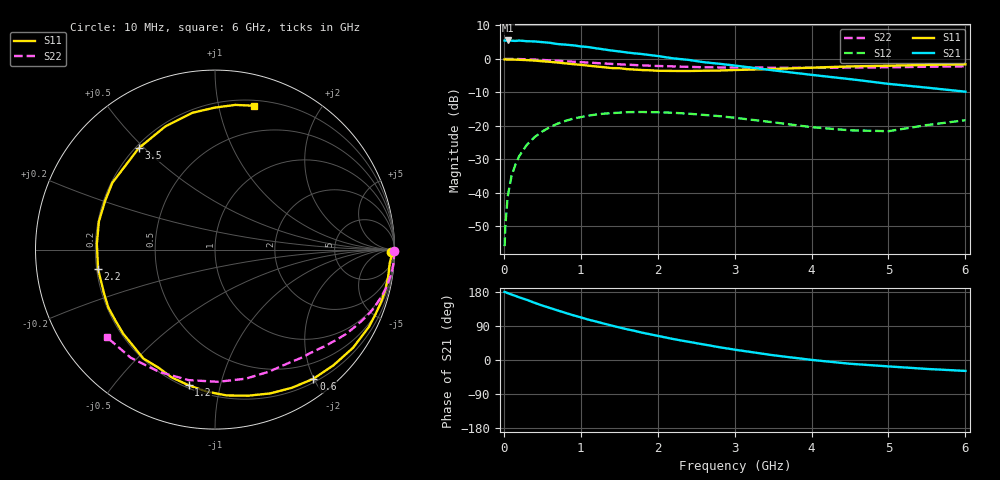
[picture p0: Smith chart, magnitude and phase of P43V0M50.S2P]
! SIEMENS Small Signal Semiconductors
! BFP182
! Si NPN RF Bipolar Junction Transistor in SOT143
! VCE = 3 V  IC = 0.5 mA
! Common Emitter S-Parameters:  March  1996
# GHz  S  MA  R  50
!  f  S11  S21  S12  S22
! GHz  MAG  ANG  MAG  ANG  MAG  ANG  MAG  ANG
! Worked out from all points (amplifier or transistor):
!   36 points, 10 MHz to 6 GHz, reference 50 ohm
!   highest |S21| = 5.5 dB at 50 MHz (marker M1)
!   |S21| within 3 dB of that: start of sweep to 1.397 GHz
!   unconditionally stable (mu >= 1): 2.983 GHz to end of sweep
!   at 250 MHz: K = 0.08, MSG = 16.3 dB, |S12| = -27.3 dB
!   at 1.4 GHz: K = 0.50, MSG = 9.3 dB, |S12| = -16.2 dB
!   at 6 GHz: K = 1.20, MAG = 1.5 dB, |S12| = -18.3 dB
!   S11 on the Smith chart (normalised r, x): 10 MHz: 69, -54; 600 MHz: 0.25, -1.99; 1.2 GHz: 0.22, -0.80; 2.2 GHz: 0.21, -0.08; 3.5 GHz: 0.21, +0.48; 6 GHz: 0.25, +1.28
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0.01  0.9822 -0.8  1.876 179.7  0.0016 91.0  0.9996 -0.3
0.02  0.9857 -1.8  1.874 179.2  0.0033 87.5  0.9985 -0.6
0.05  0.9763 -4.4  1.885 176.4  0.0088 89.0  0.9979 -1.6
0.1  0.9767 -8.8  1.873 172.8  0.0179 83.8  0.9978 -3.2
0.2  0.9701 -17.8  1.878 165.4  0.0354 78.1  0.9943 -6.4
0.3  0.9597 -26.6  1.837 158.7  0.0523 72.7  0.9858 -9.6
0.4  0.9438 -35.4  1.823 150.9  0.0681 67.0  0.9769 -12.6
0.6  0.9047 -52.7  1.738 137.3  0.0959 55.9  0.9509 -18.4
0.9  0.8347 -77.2  1.594 118.2  0.1281 41.3  0.908 -26.0
1.1  0.7925 -93.3  1.5 106.5  0.1425 32.5  0.8801 -30.6
1.2  0.7701 -101.0  1.44 101.5  0.1476 28.1  0.8674 -32.9
1.5  0.7264 -123.3  1.293 85.9  0.1574 17.5  0.8298 -38.6
1.8  0.6813 -144.4  1.18 72.0  0.1611 8.7  0.8004 -43.8
2.2  0.6606 -170.4  1.02 55.4  0.1569 -1.6  0.7731 -50.9
2.4  0.659 177.2  0.967 48.1  0.1522 -6.1  0.7603 -54.6
2.8  0.6699 156.0  0.846 33.8  0.1398 -12.7  0.7455 -61.9
3.5  0.707 127.0  0.675 12.6  0.1132 -18.9  0.7393 -76.6
4  0.7399 112.0  0.578 0.3  0.0957 -15.5  0.7368 -88.6
4.5  0.7726 99.4  0.499 -9.9  0.0859 -7.8  0.7418 -101.4
5  0.7911 90.1  0.424 -16.9  0.0833 6.9  0.7489 -114.4
5.5  0.814 82.0  0.372 -23.6  0.1029 13.9  0.7639 -127.9
6  0.8304 74.8  0.324 -28.8  0.1215 15.4  0.7748 -140.8
